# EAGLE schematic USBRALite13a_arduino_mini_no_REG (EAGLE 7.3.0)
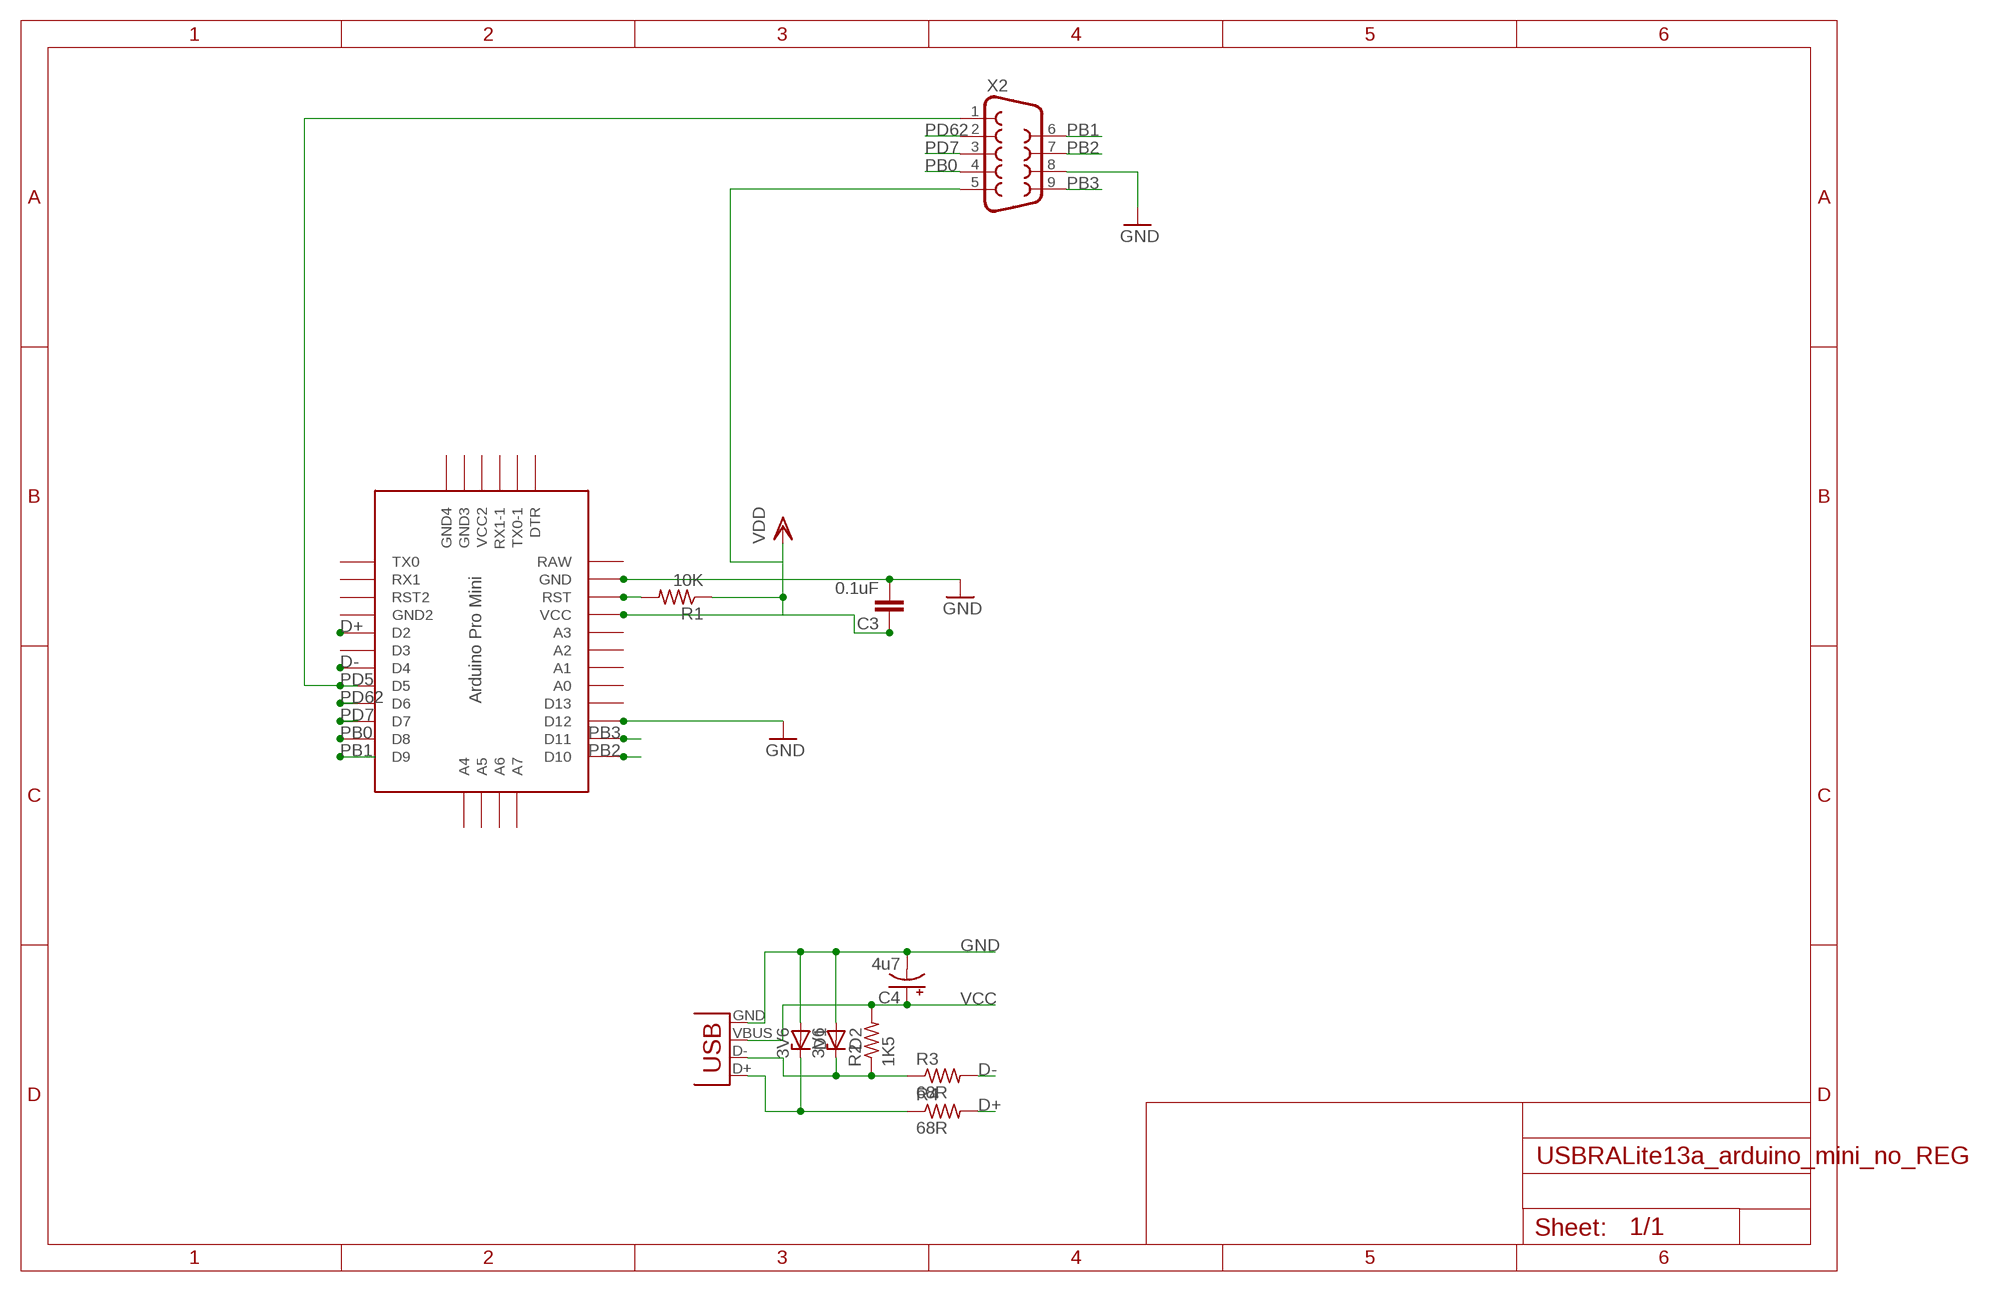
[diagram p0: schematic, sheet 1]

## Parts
C3  0.1uF  C-EU050-024X044  [C050-024X044]
C4  4u7  CPOL-USE2.5-6  [E2,5-6]
D1  3V6  ZENER-DIODEZD-5  [ZDIO-5]
D2  3V6  ZENER-DIODEZD-5  [ZDIO-5]
R1  10K  R-US_0207/10  [0207/10]
R2  1K5  R-US_0207/10  [0207/10]
R3  68R  R-US_0207/10  [0207/10]
R4  68R  R-US_0207/10  [0207/10]
U$1  PRO-MINI  [PRO-MINI]
X1  USBPTH  [USB-B-PTH]
X2  DB9MALE  [DB9_MALE]

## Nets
D+: R4.2 U$1.D2
D-: R3.2 U$1.D4
GND: C3.2 C4.- D1.A D2.A U$1.D12 U$1.GND X1.GND X2.8
N$1: R1.2 U$1.RST
N$8: D1.C R4.1 X1.D+
N$9: D2.C R2.1 R3.1 X1.D-
PB0: U$1.D8 X2.4
PB1: U$1.D9 X2.6
PB2: U$1.D10 X2.7
PB3: U$1.D11 X2.9
PD5: U$1.D5 X2.1
PD7: U$1.D7 X2.3
PD62: U$1.D6 X2.2
VCC: C3.1 C4.+ R1.1 R2.2 X1.VBUS X2.5 ; supply symbol labelled VDD
Unconnected: U$1.A0 U$1.A1 U$1.A2 U$1.A3 U$1.A4 U$1.A5 U$1.A6 U$1.A7 U$1.D3 U$1.D13 U$1.DTR U$1.GND1(GND2) U$1.GND2(GND4) U$1.GND3 U$1.RST1(RST2) U$1.RX1 U$1.RX1-1 U$1.TX0 U$1.TX0-1 U$1.VCC U$1.VCC1(VCC2)

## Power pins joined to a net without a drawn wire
RAW: U$1.RAW

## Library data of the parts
C3 = rcl:C-EU: CAPACITOR, European symbol
C4 = adafruit:CPOL-US: POLARIZED CAPACITOR, American symbol
D1 D2 = diode:ZENER-DIODE: Z-Diode
R1-R4 = adafruit:R-US_: RESISTOR, American symbol
U$1 = Arduino-clone:PRO-MINI: Arduion Pro Mini Clone V1.0 www.betemcu.cu
X1 = SparkFun:USB: USB Connectors USB-B-PTH is fully proven SKU : PRT-00139 USB-miniB is fully proven SKU : PRT-00587 USB-A-PCB is untested. USB-A-H is throughly reviewed, but untested. Spark Fun Electronics SKU : PRT-00437 USB-B-SMT is throughly reviewed, but untested. Needs silkscreen touching up. USB-A-S has not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
X2 = SparkFun:DB9: DB9 Connector Standard DB9 (D-Sub 9) serial connector. Can be used for CAN bus as well as RS485 and RS232. Footprint production proven. Spark Fun Electronics SKU : PRT-00429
